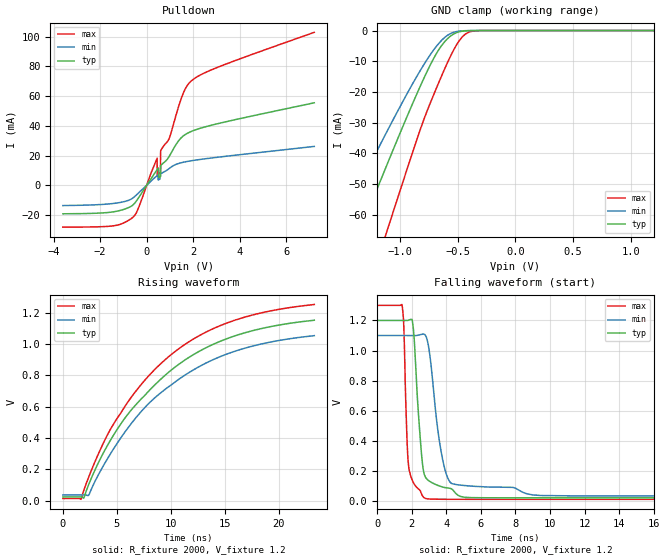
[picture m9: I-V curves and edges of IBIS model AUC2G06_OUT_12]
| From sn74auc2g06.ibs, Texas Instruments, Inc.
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[Model]   AUC2G06_OUT_12
Model_type  Open_drain
Enable   Active-Low
Vref =   0
Rref =   2000
Cref =   15p
Vmeas =   0.6
| variable   typ   min   max
C_comp   3.06pF   2.68pF   3.26pF
| C_pulldown   4.01pF   2.19pF   12.50pF
| C_tri-state   3.06pF   2.68pF   3.26pF
[Temperature Range]   40   100   -40
| Ambient temperature   25   85   -40
[Voltage range]   1.2   1.1   1.3
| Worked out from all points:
|   slope of the pulldown table from 0 to 0.18 V, typ, clamps not added: 42.4 ohm
|   GND clamp passes 1 mA (typ) near -0.53 V on its own axis
|   rising waveform, R_fixture 2000, V_fixture 1.2: 20-80 % time 8.61ns typ, 8.59ns min, 8.41ns max; typ from 0.024 V to 1.15 V
|   falling waveform, R_fixture 2000, V_fixture 1.2: 20-80 % time 416ps typ, 709ps min, 217ps max; typ from 1.2 V to 0.024 V
[GND Clamp]
| AUC2G06_OUT_12
|   Voltage   I(typ)   I(min)   I(max)
-3.6V     -279.3mA   -228.7mA   -348mA
-1.56V    -85.32mA   -66.26mA   -116.8mA
-1.51V    -80.6mA    -62.43mA   -111mA
-1.33V    -63.68mA   -48.79mA   -90.29mA
-1.125V   -44.68mA   -33.64mA   -66.54mA
-1.085V   -41.02mA   -30.76mA   -61.9mA
-825mV    -18.08mA   -12.98mA   -32.18mA
-690mV    -7.781mA   -5.339mA   -19.16mA
-570mV    -2.022mA   -1.117mA   -8.88mA
-435mV    -114.4uA   -58.08uA   -1.201mA
-315mV    -3.46uA    -2.767uA   -28.94uA
1.2V      258.8pA    425.9pA    238.4pA
[Pulldown]
| AUC2G06_OUT_12
|   Voltage   I(typ)   I(min)   I(max)
-3.6V     -19.18mA   -13.63mA   -28.17mA
-1.38V    -17.74mA   -12.12mA   -27.16mA
-535mV    -12.4mA    -7.82mA    -20.65mA
450mV     10.5mA     6.398mA    18.24mA
455mV     10.61mA    6.451mA    6.435mA
590mV     5.848mA    7.731mA    8.546mA
600mV     5.947mA    7.818mA    22.94mA
605mV     12.96mA    7.861mA    23.36mA
970mV     19.53mA    11.32mA    31.67mA
1.615V    33.73mA    15.67mA    63.55mA
1.985V    36.71mA    16.71mA    71.15mA
7.2V      55.55mA    26.19mA    103mA
[Ramp]
| AUC2G06_OUT_12
| variable   typ   min   max
dV/dt_r   0.68/8.62E-09   0.61/8.59E-09   0.75/8.41E-09
dV/dt_f   0.71/4.23E-10   0.64/7.15E-10   0.78/2.33E-10
R_load = 2000
[Rising Waveform]
| AUC2G06_OUT_12
R_fixture =   2000
C_fixture =   0
L_fixture =   0
V_fixture =   1.2
V_fixture_min = 1.1
V_fixture_max = 1.3
|   Time   V(typ)   V(min)   V(max)
0s        23.98mV    36.64mV    13.86mV
1.69ns    23.87mV    36.6mV     8.747mV
1.945ns   18.04mV    36.42mV    66.72mV
2.395ns   102.7mV    35.94mV    150.7mV
4.16ns    355.9mV    270.8mV    424mV
6.005ns   550.5mV    462mV      628.2mV
8.04ns    705.8mV    625.9mV    803.3mV
10.39ns   852.4mV    757.2mV    951.8mV
15.85ns   1.05V      951.8mV    1.15V
23.3ns    1.152V     1.054V     1.252V
[Falling Waveform]
| AUC2G06_OUT_12
R_fixture =   2000
C_fixture =   0
L_fixture =   0
V_fixture =   1.2
V_fixture_min = 1.1
V_fixture_max = 1.3
|   Time   V(typ)   V(min)   V(max)
0s        1.2V       1.1V       1.3V
1.435ns   1.2V       1.1V       1.304V
1.535ns   1.2V       1.1V       1.179V
1.765ns   1.2V       1.1V       314.7mV
2.015ns   1.207V     1.1V       144.9mV
2.545ns   342.8mV    1.107V     56.29mV
2.78ns    164mV      1.103V     20.73mV
3.71ns    98.11mV    324.7mV    14.35mV
4.31ns    82.67mV    118.9mV    14mV
23.3ns    23.98mV    36.65mV    13.86mV
